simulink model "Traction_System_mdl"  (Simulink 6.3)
settings: Solver=ode45  StartTime=0.0  StopTime=10.0  RelTol=1e-6  AbsTol=1e-6
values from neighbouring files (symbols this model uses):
  a_res = 1    [Traction_System.m]
  alpha = 0    [Traction_System.m]
  b_res = 2    [Traction_System.m]
  Bg = ones(3,1)    [Traction_System.m]
  C_f = 200*microF    (= 0.0002)    [Traction_System.m]
  g = 9.81*metri/(sec^2)    (= 9.81)    [Traction_System.m]
  i_filter_0 = 0*Amp    (= 0)    [Traction_System.m]
  I_M_0 = [i_field1_0 i_arm i_field2_0]    [Traction_System.m]
  k_mach1 = 0.1    [Traction_System.m]
  k_mach2 = 0.1    [Traction_System.m]
  L_f = 20*mH    (= 0.02)    [Traction_System.m]
  L_M = diag([L_field1 L_arm1+L_arm2 L_field2])    [Traction_System.m]
  M = 10000*kg    (= 10000)    [Traction_System.m]
  M_b = [mbog1 mbog2]    [Traction_System.m]
  m_chop = [0.3 0.9 0.3]    [Traction_System.m]
  m_chop_phase = [0 0.33 0.66]    [Traction_System.m]
  R_f = 2*Ohm    (= 2)    [Traction_System.m]
  R_M = diag([R_field1 R_arm1+R_arm2 R_field2])    [Traction_System.m]
  Tc = Ts/50    (= 4e-07)    [Traction_System.m]
  Ts = 0.02*msec    (= 2e-05)    [Traction_System.m]
  u_filter_0 = 0*Volt    (= 0)    [Traction_System.m]
  V_DC = 400*Volt    (= 400)    [Traction_System.m]
  v_sub_0 = 30*km/ora    (= 8.33333333333)    [Traction_System.m]
libraries: simulink x1

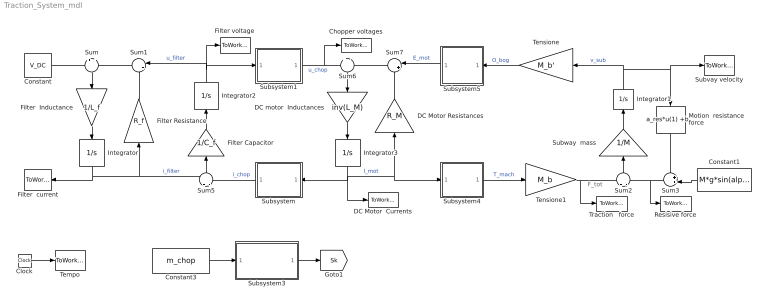
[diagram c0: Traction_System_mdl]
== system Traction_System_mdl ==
  note: F_tot
  Chopper voltages : ToWorkspace  VariableName=u_chop  SampleTime=Tc  SaveFormat=Array
  Clock : Clock
  Constant : Constant  Value=V_DC
  Constant1 : Constant  Orientation=left  Value=M*g*sin(alpha)
  Constant3 : Constant  Value=m_chop
  DC Motor Resistances : Gain  Orientation=up  Gain=R_M  Multiplication=Matrix(K*u) (u vector)
  DC Motor  Currents : ToWorkspace  VariableName=I_mot  SampleTime=Tc  SaveFormat=Array
  DC motor  Inductances : Gain  Orientation=down  Gain=inv(L_M)  Multiplication=Matrix(K*u) (u vector)
  Filter Capacitor : Gain  Orientation=up  Gain=1/C_f
  Filter Resistance : Gain  Orientation=up  Gain=R_f
  Filter voltage : ToWorkspace  VariableName=u_filter  SampleTime=Tc  SaveFormat=Array
  Filter  Inductance : Gain  Orientation=down  Gain=1/L_f
  Filter  current : ToWorkspace  VariableName=i_filter  SampleTime=Tc  SaveFormat=Array
  Integrator : Integrator  Orientation=down  InitialCondition=i_filter_0  LowerSaturationLimit=0
  Integrator1 : Integrator  Orientation=up  InitialCondition=v_sub_0
  Integrator2 : Integrator  Orientation=up  InitialCondition=u_filter_0
  Integrator3 : Integrator  Orientation=down  InitialCondition=I_M_0  LowerSaturationLimit=0
  Motion  resistance force : Fcn  Orientation=down  Expr=a_res*u(1) +b_res*u(1)*abs(u(1))
  Resisive force : ToWorkspace  VariableName=F_res  SampleTime=Tc  SaveFormat=Array
  Subsystem : Subsystem  Orientation=left
  Subsystem1 : Subsystem
  Subsystem3 : Subsystem
  Subsystem4 : Subsystem
  Subsystem5 : Subsystem  Orientation=left
  Subvay velocity : ToWorkspace  VariableName=v_sub  SampleTime=Tc  SaveFormat=Array
  Subway  mass : Gain  Orientation=up  Gain=1/M
  Sum : Sum  Orientation=down  Inputs=+|-
  Sum1 : Sum  Orientation=left  Inputs=|++
  Sum2 : Sum  Orientation=up  Inputs=+|-
  Sum3 : Sum  Orientation=left  Inputs=++|
  Sum5 : Sum  Orientation=up  Inputs=+|-
  Sum6 : Sum  Orientation=down  Inputs=+|-
  Sum7 : Sum  Orientation=left  Inputs=|++
  Tempo : ToWorkspace  VariableName=t  SampleTime=Tc  SaveFormat=Array
  Tensione : Gain  Orientation=left  Gain=M_b'  Multiplication=Matrix(K*u) (u vector)
  Tensione1 : Gain  Gain=M_b  Multiplication=Matrix(K*u) (u vector)
  Traction   force : ToWorkspace  VariableName=F_tot  SampleTime=Tc  SaveFormat=Array
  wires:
  Clock/1 -> Tempo/1
  Sum/1 -> Filter  Inductance/1
  Filter  Inductance/1 -> Integrator/1
  Integrator/1 -> Filter Resistance/1, Sum5/1, Filter  current/1  "i_filter"
  Sum1/1 -> Sum/2
  Filter Resistance/1 -> Sum1/2
  Sum2/1 -> Subway  mass/1
  Subway  mass/1 -> Integrator1/1
  Integrator1/1 -> Subvay velocity/1, Motion  resistance force/1, Tensione/1  "v_sub"
  Motion  resistance force/1 -> Sum3/1
  Sum3/1 -> Sum2/2, Resisive force/1
  Constant1/1 -> Sum3/2
  Constant/1 -> Sum/1
  Tensione1/1 -> Sum2/1, Traction   force/1
  Sum5/1 -> Filter Capacitor/1
  Filter Capacitor/1 -> Integrator2/1
  Subsystem/1(Out1) -> Sum5/2  "i_chop"
  Integrator2/1 -> Sum1/1, Subsystem1/1(In1), Filter voltage/1  "u_filter"
  Sum6/1 -> DC motor  Inductances/1
  DC motor  Inductances/1 -> Integrator3/1
  Integrator3/1 -> DC Motor  Currents/1, Subsystem4/1(In1), DC Motor Resistances/1, Subsystem/1(In1)  "I_mot"
  Sum7/1 -> Sum6/2
  DC Motor Resistances/1 -> Sum7/2
  Subsystem1/1(Out1) -> Sum6/1, Chopper voltages/1  "u_chop"
  Subsystem5/1(Out1) -> Sum7/1  "E_mot"
  Subsystem4/1(Out1) -> Tensione1/1  "T_mach"
  Tensione/1 -> Subsystem5/1(In1)  "O_bog"
  Subsystem3/1(Out1) -> [Sk]
  Constant3/1 -> Subsystem3/1(In1)

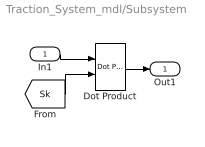
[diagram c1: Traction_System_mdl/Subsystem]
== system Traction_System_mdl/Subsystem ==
  In1 : Inport
  Dot Product : simulink/Math Operations/Dot Product  InputSameDT=on  OutDataType=sfix(16)  OutScaling=2^-10  DoSatur=off
  Out1 : Outport
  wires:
  [Sk] -> Dot Product/2
  In1/1 -> Dot Product/1
  Dot Product/1 -> Out1/1

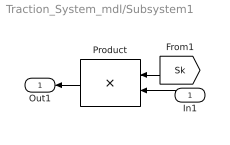
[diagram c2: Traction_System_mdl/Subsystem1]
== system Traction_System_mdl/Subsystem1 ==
  In1 : Inport  Orientation=left
  Product : Product  Orientation=left  Multiplication=Matrix(*)
  Out1 : Outport  Orientation=left
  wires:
  [Sk] -> Product/1
  In1/1 -> Product/2
  Product/1 -> Out1/1

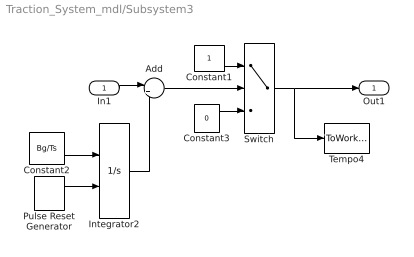
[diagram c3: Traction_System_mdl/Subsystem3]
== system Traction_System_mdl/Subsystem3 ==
  In1 : Inport
  Add : Sum  Inputs=|+-  OutScaling=2^-10
  Constant1 : Constant
  Constant2 : Constant  Value=Bg/Ts
  Constant3 : Constant  Value=0
  Integrator2 : Integrator  ExternalReset=rising
  Pulse Reset Generator : DiscretePulseGenerator  PulseType=Time based  Period=Ts  PulseWidth=50  PhaseDelay=m_chop_phase*Ts
  Switch : Switch
  Tempo4 : ToWorkspace  VariableName=Sk  SampleTime=Tc  SaveFormat=Array
  Out1 : Outport
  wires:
  Pulse Reset Generator/1 -> Integrator2/2
  Constant2/1 -> Integrator2/1
  Integrator2/1 -> Add/2
  Add/1 -> Switch/2
  Switch/1 -> Tempo4/1, Out1/1
  In1/1 -> Add/1
  Constant1/1 -> Switch/1
  Constant3/1 -> Switch/3

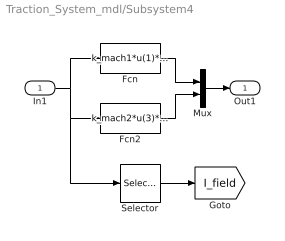
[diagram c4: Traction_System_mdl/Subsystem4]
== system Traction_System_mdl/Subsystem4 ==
  In1 : Inport
  Fcn : Fcn  Expr=k_mach1*u(1)*u(2)
  Fcn2 : Fcn  Expr=k_mach2*u(3)*u(2)
  Mux : Mux  Inputs=2
  Selector : Selector  Elements=[1 3]  InputPortWidth=3
  Out1 : Outport
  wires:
  Fcn/1 -> Mux/1
  Fcn2/1 -> Mux/2
  In1/1 -> Fcn/1, Fcn2/1, Selector/1
  Mux/1 -> Out1/1
  Selector/1 -> [I_field]

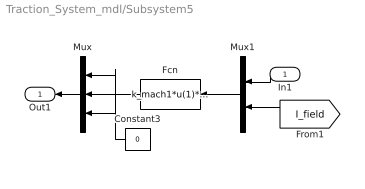
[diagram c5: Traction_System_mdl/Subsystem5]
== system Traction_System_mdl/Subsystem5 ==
  In1 : Inport  Orientation=left
  Constant3 : Constant  Orientation=left  Value=0
  Fcn : Fcn  Orientation=left  Expr=k_mach1*u(1)*u(3)+k_mach2*u(2)*u(4)
  Mux : Mux  Orientation=left  Inputs=3
  Mux1 : Mux  Orientation=left  Inputs=2
  Out1 : Outport  Orientation=left
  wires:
  [I_field] -> Mux1/2
  Mux1/1 -> Fcn/1
  Fcn/1 -> Mux/2
  Constant3/1 -> Mux/1, Mux/3
  In1/1 -> Mux1/1
  Mux/1 -> Out1/1
